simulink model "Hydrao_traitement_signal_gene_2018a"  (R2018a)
settings: Solver=VariableStepAuto  StartTime=0.0  StopTime=3  RelTol=1e-3

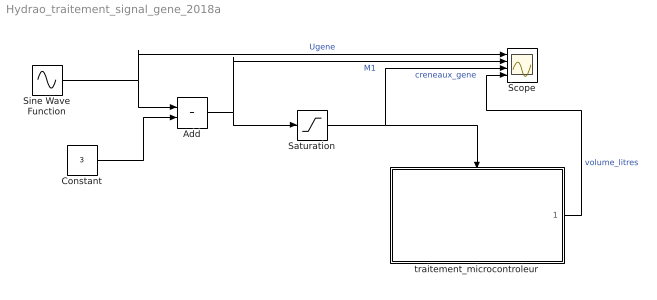
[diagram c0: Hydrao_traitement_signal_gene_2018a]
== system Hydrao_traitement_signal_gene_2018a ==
  Add : Sum
  Constant : Constant  Value=3
  Saturation : Saturate  UpperLimit=3  LowerLimit=0
  Scope : Scope  NumInputPorts=4
  Sine Wave Function : Sin  Amplitude=4  Frequency=10*2*pi  SampleTime=0.001
  traitement_microcontroleur : Stateflow chart  TreatAsAtomicUnit=on
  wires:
  Sine Wave Function/1 -> Add/1, Scope/1  "Ugene"
  Constant/1 -> Add/2
  Add/1 -> Saturation/1, Scope/2  "M1"
  Saturation/1 -> traitement_microcontroleur/Trigger, Scope/3  "creneaux_gene"
  traitement_microcontroleur/1(volume) -> Scope/4  "volume_litres"

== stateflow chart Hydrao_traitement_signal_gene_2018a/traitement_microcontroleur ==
  state cumul_volume
    en : volume=volume+1/545
  (default) -> cumul_volume : {volume=0}
  cumul_volume -> cumul_volume : tour
  data: volume output
  events: input RISING_EDGE_EVENT
